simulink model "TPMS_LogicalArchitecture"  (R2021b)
settings: Solver=VariableStepAuto  StartTime=0.0  StopTime=10.0  RelTol=1e-3

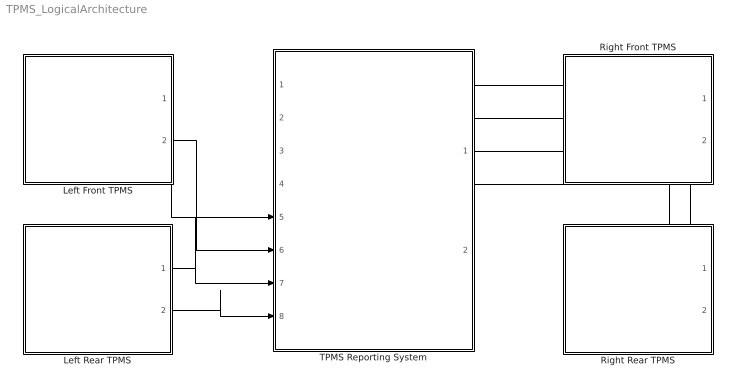
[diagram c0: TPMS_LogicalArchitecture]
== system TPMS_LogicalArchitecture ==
  Left Front TPMS : ModelReference  ModelNameDialog=TPMS  SimulationMode=Normal  ModelReferenceVersion=1.12
  Left Rear TPMS : ModelReference  ModelNameDialog=TPMS  SimulationMode=Normal  ModelReferenceVersion=1.12
  Right Front TPMS : ModelReference  ModelNameDialog=TPMS  SimulationMode=Normal  ModelReferenceVersion=1.12
  Right Rear TPMS : ModelReference  ModelNameDialog=TPMS  SimulationMode=Normal  ModelReferenceVersion=1.12
  TPMS Reporting System : Subsystem
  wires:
  Left Front TPMS/1 -> TPMS Reporting System/5(isTirePressureLow1)
  Left Front TPMS/2 -> TPMS Reporting System/6(calibTirePressure1)
  Left Rear TPMS/1 -> TPMS Reporting System/7(Bus Element In3)
  Left Rear TPMS/2 -> TPMS Reporting System/8(Bus Element In4)
  Right Front TPMS/1 -> TPMS Reporting System/1(isTirePressureLow2)
  Right Front TPMS/2 -> TPMS Reporting System/2(calibTirePressure2)
  Right Rear TPMS/1 -> TPMS Reporting System/3(isTirePressureLow3)
  Right Rear TPMS/2 -> TPMS Reporting System/4(calibTirePressure3)

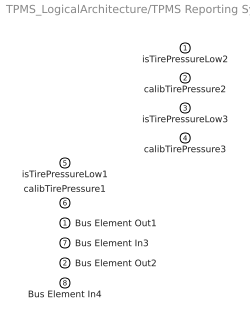
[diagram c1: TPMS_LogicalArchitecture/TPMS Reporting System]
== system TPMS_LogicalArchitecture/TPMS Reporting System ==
  isTirePressureLow2 : Inport
  calibTirePressure2 : Inport  Port=2
  isTirePressureLow3 : Inport  Port=3
  calibTirePressure3 : Inport  Port=4
  isTirePressureLow1 : Inport  Port=5
  calibTirePressure1 : Inport  Port=6
  Bus Element In3 : Inport  Port=7
  Bus Element In4 : Inport  Port=8
  Bus Element Out1 : Outport
  Bus Element Out2 : Outport  Port=2
